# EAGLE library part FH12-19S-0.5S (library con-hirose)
0.5mm Pitch Connectors For FPC/FFC Source: Data sheet
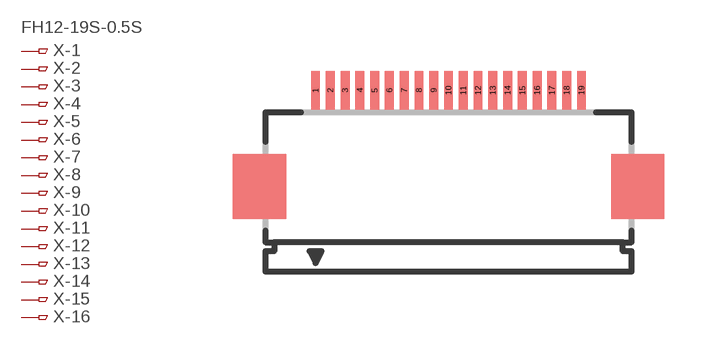
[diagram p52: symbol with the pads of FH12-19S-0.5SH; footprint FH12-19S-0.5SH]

Designator prefix X; gates -1=PINV -2=PIN -3=PIN -4=PIN -5=PIN -6=PIN -7=PIN -8=PIN -9=PIN -10=PIN -11=PIN -12=PIN -13=PIN -14=PIN -15=PIN -16=PIN -17=PIN -18=PIN -19=PIN

## FH12-19S-0.5SH (OC_FARNELL: unknown; OC_NEWARK: unknown)  [FH12-19S-0.5SH]
1  -1:1  pas
2  -2:1  pas
3  -3:1  pas
4  -4:1  pas
5  -5:1  pas
6  -6:1  pas
7  -7:1  pas
8  -8:1  pas
9  -9:1  pas
10  -10:1  pas
11  -11:1  pas
12  -12:1  pas
13  -13:1  pas
14  -14:1  pas
15  -15:1  pas
16  -16:1  pas
17  -17:1  pas
18  -18:1  pas
19  -19:1  pas

## Footprint FH12-19S-0.5SH (pad centres in mm)
0.5mm Pitch Connectors For FPC/FFC Source: Data sheet
smd 0.3 x 1.3: 1 -4.5,3.25; 2 -4,3.25; 3 -3.5,3.25; 4 -3,3.25; 5 -2.5,3.25; 6 -2,3.25; 7 -1.5,3.25; 8 -1,3.25; 9 -0.5,3.25; 10 0,3.25; 11 0.5,3.25; 12 1,3.25; 13 1.5,3.25; 14 2,3.25; 15 2.5,3.25; 16 3,3.25; 17 3.5,3.25; 18 4,3.25; 19 4.5,3.25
